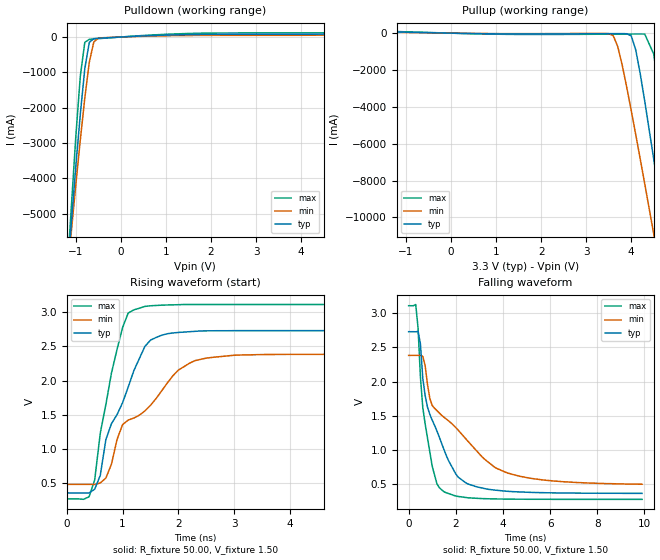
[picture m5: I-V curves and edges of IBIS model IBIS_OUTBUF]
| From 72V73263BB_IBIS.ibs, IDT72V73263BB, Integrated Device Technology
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|   Model IBIS_OUTBUF
[Model]   IBIS_OUTBUF
Model_type   Output
Polarity   Non-Inverting
Enable   Active-High
Vinl =  0.000V
Vinh =  3.300V
Vmeas =  1.500V
Cref = 30.000pF
Rref = 50.000
Vref =  1.500V
C_comp   3.00pF   2.00pF   4.00pF
[Temperature Range]   25.00   85.00   -40.00
[Voltage Range]   3.30V   3.00V   3.60V
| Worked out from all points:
|   slope of the pulldown table from 0 to 0.495 V, typ, clamps not added: 16.1 ohm
|   slope of the pullup table from 0 to 0.495 V, typ, clamps not added: 22.5 ohm
|   rising waveform, R_fixture 50.00, V_fixture 1.50: 20-80 % time 621ps typ, 1.01ns min, 385ps max; typ from 0.355 V to 2.73 V
|   falling waveform, R_fixture 50.00, V_fixture 1.50: 20-80 % time 1.14ns typ, 2.4ns min, 527ps max; typ from 2.73 V to 0.356 V
[Pulldown]
| voltage   I(typ)   I(min)   I(max)
-3.3V     -42.01A    -36.04A    -50.9A
-1.5V     -11.71A    -10.89A    -12.87A
-1V       -3.67A     -4.184A    -2.828A
-900mV    -2.19A     -2.919A    -1.111A
-800mV    -893.8mA   -1.729A    -150.1mA
-700mV    -151.7mA   -712.2mA   -66.26mA
-600mV    -46.32mA   -137.8mA   -55.05mA
-500mV    -34.57mA   -33.64mA   -46mA
-400mV    -27.67mA   -20.48mA   -37.18mA
1.5V      67.91mA    43.34mA    99.95mA
4.7V      84.5mA     56.12mA    122mA
6.6V      131mA      78.82mA    191mA
[Pullup]
| voltage   I(typ)   I(min)   I(max)
-3.3V     37.98mA    18.68mA    52.21mA
3.5V      -28.52mA   -25.59mA   -54.78mA
3.6V      -27.26mA   -135mA     -53.29mA
3.7V      -26.03mA   -719mA     -51.79mA
4V        -146mA     -4.195A    -47.34mA
4.1V      -906mA     -5.501A    -45.99mA
4.3V      -3.69A     -8.177A    -48.91mA
4.5V      -6.84A     -10.9A     -1.137A
4.7V      -10.09A    -13.65A    -4.78A
4.9V      -13.39A    -16.42A    -8.799A
5.1V      -16.72A    -19.2A     -12.91A
6.6V      -42.01A    -40.27A    -44.53A
[Ramp]
| variable   typ   min   max
dV/dt_r   1.24/0.78n   0.81/1.40n   1.61/0.41n
dV/dt_f   1.46/1.40n   1.11/2.62n   1.74/0.72n
R_load = 50.00
[Rising Waveform]
R_fixture = 50.00
V_fixture = 1.50
C_fixture = 0.000F
| time   V(typ)   V(min)   V(max)
0s        355mV      480mV      268mV
400ps     355mV      480mV      299mV
500ps     409mV      479mV      545mV
600ps     611mV      500mV      1.229V
700ps     1.135V     572mV      1.648V
900ps     1.501V     1.136V     2.455V
1.2ns     2.142V     1.451V     3.035V
1.5ns     2.592V     1.638V     3.095V
2.5ns     2.728V     2.329V     3.114V
9.9ns     2.731V     2.384V     3.114V
[Falling Waveform]
R_fixture = 50.00
V_fixture = 1.50
C_fixture = 0.000F
| time   V(typ)   V(min)   V(max)
0s        2.732V     2.384V     3.114V
300ps     2.731V     2.384V     3.132V
400ps     2.738V     2.384V     2.784V
500ps     2.554V     2.386V     2.064V
700ps     1.793V     2.234V     1.378V
1ns       1.431V     1.647V     756mV
1.5ns     998mV      1.474V     379mV
2.4ns     517mV      1.167V     296mV
4.2ns     386mV      654mV      271mV
9.9ns     356mV      490mV      268mV
